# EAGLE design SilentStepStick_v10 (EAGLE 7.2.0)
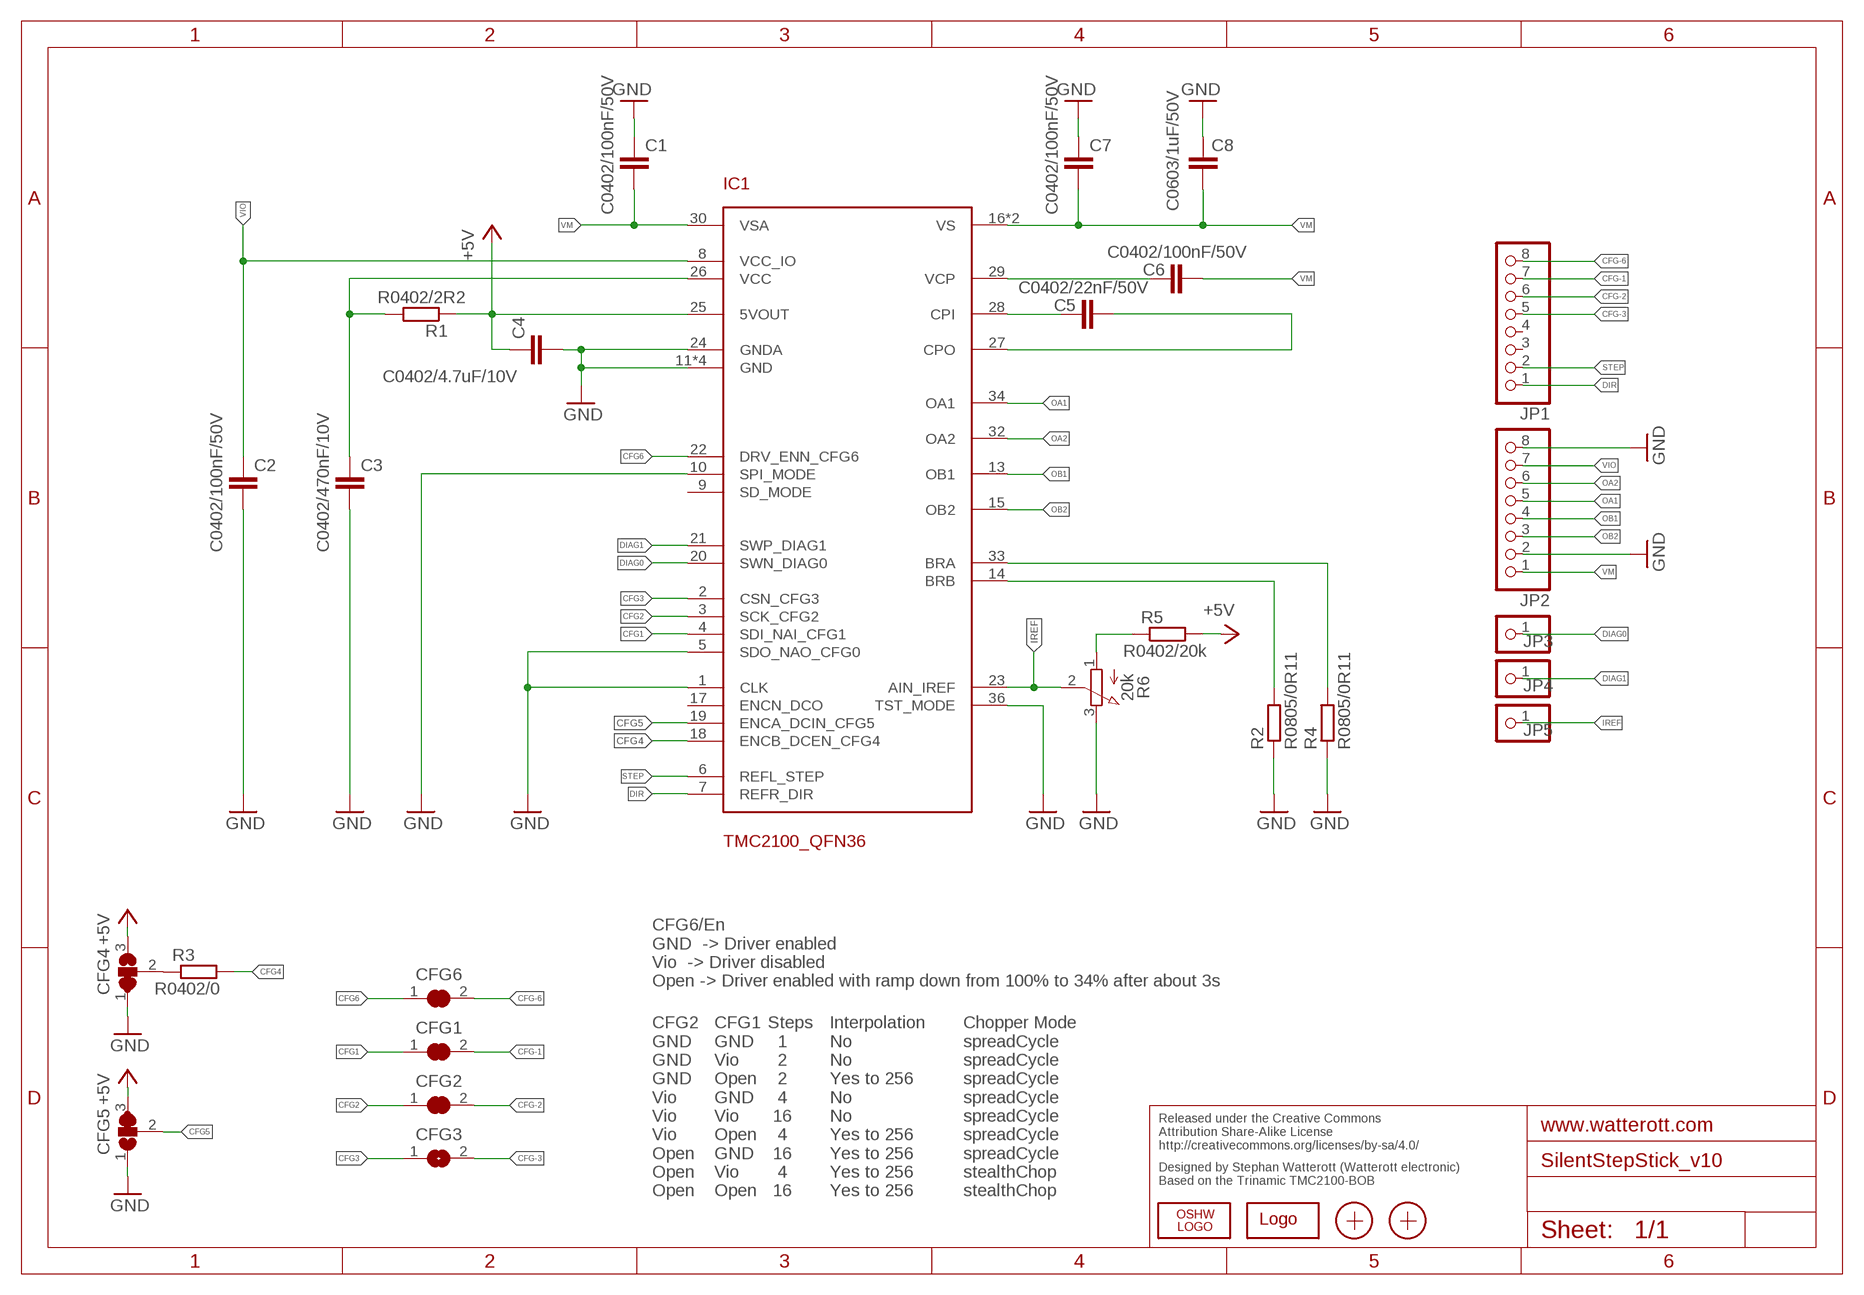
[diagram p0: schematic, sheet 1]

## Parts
C1  C0402/100nF/50V  C-EUC0402  [C0402]
C2  C0402/100nF/50V  C-EUC0402  [C0402]
C3  C0402/470nF/10V  C-EUC0402  [C0402]
C4  C0402/4.7uF/10V  C-EUC0402  [C0402]
C5  C0402/22nF/50V  C-EUC0402  [C0402]
C6  C0402/100nF/50V  C-EUC0402  [C0402]
C7  C0402/100nF/50V  C-EUC0402  [C0402]
C8  C0603/1uF/50V  C-EUC0603  [C0603]
CFG1  JUMPER2-0201  [JUMPER2-0201]
CFG2  JUMPER2-0201  [JUMPER2-0201]
CFG3  JUMPER2-0201  [JUMPER2-0201]
CFG4  JUMPER3-0201-NC  [JUMPER3-0201_NC]
CFG5  JUMPER3-0201  [JUMPER3-0201]
CFG6  JUMPER2-0201  [JUMPER2-0201]
IC1  TMC2100_QFN36  [QFN36]
JP1  PINHD-1X08_2.54-S  [1X08-S]
JP2  PINHD-1X08_2.54-S  [1X08-S]
JP3  PINHD-1X1  [1X01]
JP4  PINHD-1X1  [1X01]
JP5  PINHD-1X1  [1X01]
LOGO1  OSHW_LOGOX0070  [OSHW_6X70]
LOGO2  LOGO-S_PLACE_M  [SPARK_TPLACE_M]
R1  R0402/2R2  R-EU_R0402  [R0402]
R2  R0805/0R11  R-EU_M0805  [M0805]
R3  R0402/0  R-EU_R0402  [R0402]
R4  R0805/0R11  R-EU_M0805  [M0805]
R5  R0402/20k  R-EU_R0402  [R0402]
R6  20k  POTEVM3R  [POT_EVM3R]
X1  PASSER-07  [PASSER_07MM]
X2  PASSER-07  [PASSER_07MM]

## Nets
+5V: C4.1 CFG4.3 CFG5.3 IC1.25(5VOUT) R1.1 R5.2
CFG1: CFG1.1 IC1.4(SDI_NAI_CFG1)
CFG2: CFG2.1 IC1.3(SCK_CFG2)
CFG3: CFG3.1 IC1.2(CSN_CFG3)
CFG4: IC1.18(ENCB_DCEN_CFG4) R3.2
CFG5: CFG5.2 IC1.19(ENCA_DCIN_CFG5)
CFG6: CFG6.1 IC1.22(DRV_ENN_CFG6)
CFG-1: CFG1.2 JP1.7
CFG-2: CFG2.2 JP1.6
CFG-3: CFG3.2 JP1.5
CFG-6: CFG6.2 JP1.8
CPI: C5.1 IC1.28(CPI)
CPO: C5.2 IC1.27(CPO)
DIAG0: IC1.20(SWN_DIAG0) JP3.1
DIAG1: IC1.21(SWP_DIAG1) JP4.1
DIR: IC1.7(REFR_DIR) JP1.1
GND: C1.1 C2.2 C3.2 C4.2 C7.1 C8.2 CFG4.1 CFG5.1 IC1.1(CLK) IC1.5(SDO_NAO_CFG0) IC1.10(SPI_MODE) IC1.11(GND) IC1.12(GND) IC1.24(GNDA) IC1.35(GND) IC1.36(TST_MODE) IC1.GND_PAD(GND) JP2.2 JP2.8 R2.1 R4.1 R6.3(E)
IREF: IC1.23(AIN_IREF) JP5.1 R6.2(S)
N$1: CFG4.2 R3.1
N$7: IC1.33(BRA) R4.2
N$9: IC1.14(BRB) R2.2
OA1: IC1.34(OA1) JP2.5
OA2: IC1.32(OA2) JP2.6
OB1: IC1.13(OB1) JP2.4
OB2: IC1.15(OB2) JP2.3
STEP: IC1.6(REFL_STEP) JP1.2
VCC: C3.1 IC1.26(VCC) R1.2
VCP: C6.1 IC1.29(VCP)
VIO: C2.1 IC1.8(VCC_IO) JP2.7
VM: C1.2 C6.2 C7.2 C8.1 IC1.16(VS) IC1.30(VSA) IC1.31(VS) JP2.1
VREF1: R5.1 R6.1(A)
Unconnected: IC1.9(SD_MODE) IC1.17(ENCN_DCO) JP1.3 JP1.4

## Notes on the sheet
- CFG6/En
  GND  -> Driver enabled
  Vio  -> Driver disabled
  Open -> Driver enabled with ramp down from 100% to 34% after about 3s
- CFG2
  GND
  GND
  GND
  Vio
  Vio
  Vio
  Open
  Open
  Open
- CFG1
  GND
  Vio
  Open
  GND
  Vio
  Open
  GND
  Vio
  Open
- Steps
    1
    2
    2
    4
   16
    4
   16
    4
   16
- Interpolation
  No
  No
  Yes to 256
  No
  No
  Yes to 256
  Yes to 256
  Yes to 256
  Yes to 256
- Chopper Mode
  spreadCycle
  spreadCycle
  spreadCycle
  spreadCycle
  spreadCycle
  spreadCycle
  spreadCycle
  stealthChop
  stealthChop
- Released under the Creative Commons
  Attribution Share-Alike License
  http://creativecommons.org/licenses/by-sa/4.0/
- Designed by Stephan Watterott (Watterott electronic) 
  Based on the Trinamic TMC2100-BOB

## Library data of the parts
C1-C8 = rcl:C-EU: CAPACITOR, European symbol
CFG1-CFG3 CFG6 = we-rcl:JUMPER2: 2 Pin Jumpers
CFG4 CFG5 = we-rcl:JUMPER3: 3 Pin Jumpers
IC1 = TMC2100_QFN:TMC2100_QFN36
JP1 JP2 = pinhead-2:PINHD-1X08: PIN HEADER
JP3-JP5 = pinhead:PINHD-1X1: PIN HEADER
LOGO1 = we-symbol:OSHW_LOGO: Open-Source-Hardware Logo
LOGO2 = we-symbol:LOGO: Watterott electronic Logo
R1-R5 = rcl:R-EU_: RESISTOR, European symbol
R6 = we-rcl:POT: Potentiometer
X1 X2 = we-symbol:PASSER: Fiducial Markers

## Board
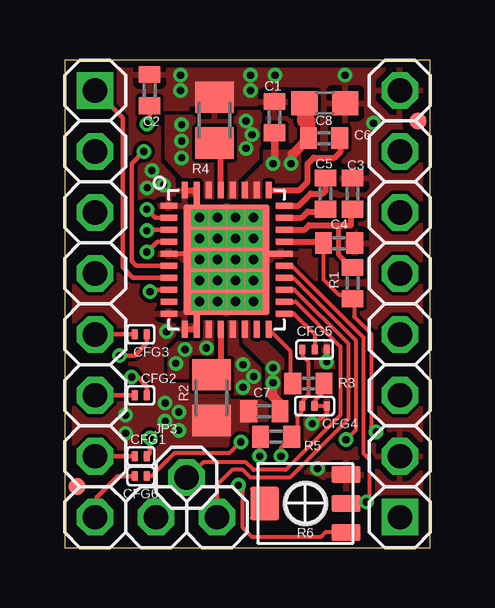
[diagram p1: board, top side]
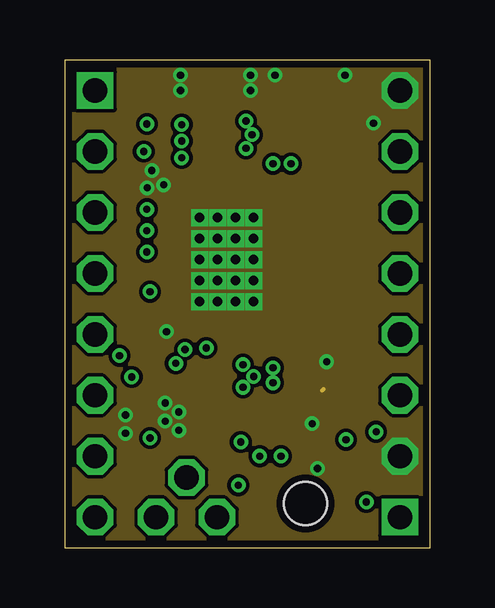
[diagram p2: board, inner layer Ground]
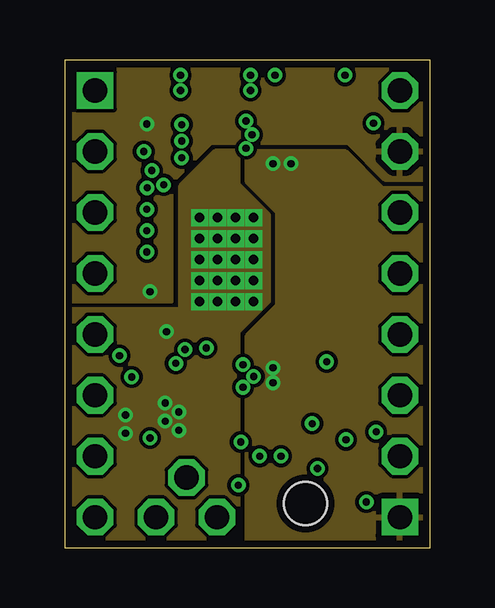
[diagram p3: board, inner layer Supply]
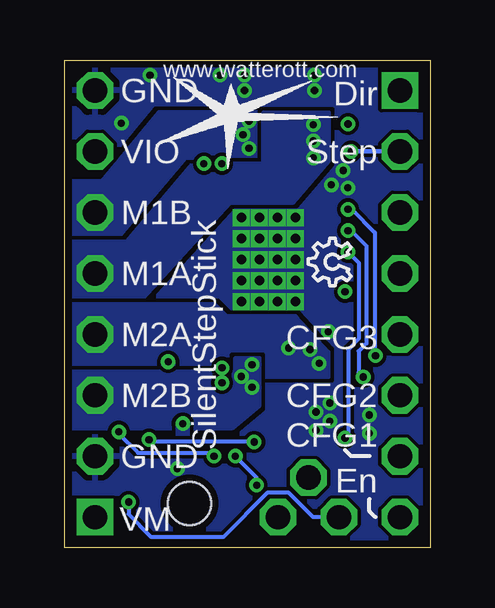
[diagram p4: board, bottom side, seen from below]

Size 15.24 x 20.32 mm. Coordinates in mm from the lower left corner, seen from the top.
Outline: 0,0 15.24,0 15.24,20.32 0,20.32 0,0
Copper layers (1*2*15*16): Top 0.035mm / dielectric 0.36mm / Ground 0.035mm / dielectric 0.71mm / Supply 0.035mm / dielectric 0.2mm / Bottom 0.035mm
Design rules "Default_WE_Euro *": minimum track width 0.15mm, minimum drill 0.25mm, track to track 0.15mm, track to pad 0.15mm, pad to pad 0.15mm, via to via 0.15mm, smd to smd 0mil, copper to edge 0.3mm, drill to drill 8mil, minimum pad ring 10mil, minimum via ring 6mil, stop-mask expansion 2mil, vias tented up to drill 0.35mm, thermal gap 10mil

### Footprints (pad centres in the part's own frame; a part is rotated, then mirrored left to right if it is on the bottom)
C0402 = smd 0.7 x 0.9: 1 -0.65,0; 2 0.65,0
C0603 = smd 1.1 x 1: 1 -0.85,0; 2 0.85,0
JUMPER2-0201 = smd 0.43 x 0.28: 1 0,0.255; 2 0,-0.255
JUMPER3-0201_NC = smd 0.43 x 0.28: 1 0,0.509; 2 0,-0.001; 3 0,-0.509
JUMPER3-0201 = smd 0.43 x 0.28: 1 0,0.51; 2 0,0; 3 0,-0.51
QFN36 = smd 0.7 x 0.25: 1 -2.4,2.25; 2 -2.4,1.75; 3 -2.4,1.25; 4 -2.4,0.75; 5 -2.4,0.25; 6 -2.4,-0.25; 7 -2.4,-0.75; 8 -2.4,-1.25; 9 -2.4,-1.75; 10 -2.4,-2.25; 19 2.4,-2.25; 20 2.4,-1.75; 21 2.4,-1.25; 22 2.4,-0.75; 23 2.4,-0.25; 25 2.4,0.75; 26 2.4,1.25; 27 2.4,1.75; 28 2.4,2.25 | smd 0.25 x 0.7: 11 -1.75,-2.9; 13 -0.75,-2.9; 14 -0.25,-2.9; 15 0.25,-2.9; 16 0.75,-2.9; 17 1.25,-2.9; 18 1.75,-2.9; 29 1.75,2.9; 30 1.25,2.9; 31 0.75,2.9; 32 0.25,2.9; 33 -0.25,2.9; 34 -0.75,2.9; 36 -1.75,2.9 | smd 0.25 x 1: 12 -1.25,-2.75; 35 -1.25,2.75 | smd 1 x 0.25: 24 2.25,0.25 | smd 3.6 x 4.6: GND_PAD 0,0
1X08-S = drill 1.016 square: 1 -8.89,0 | drill 1.016 octagon: 2 -6.35,0; 3 -3.81,0; 4 -1.27,0; 5 1.27,0; 6 3.81,0; 7 6.35,0; 8 8.89,0
1X01 = drill 1.016 octagon: 1 0,0
R0402 = smd 0.7 x 0.9: 1 -0.65,0; 2 0.65,0
M0805 = smd 1.3 x 1.6: 1 -0.95,0; 2 0.95,0
POT_EVM3R = smd 0.7 x 1.2: 1 -1.2,-1.7; 2 0,-1.7; 3 1.2,-1.7 | smd 1.4 x 1.2: MOUNT 0,1.7 | hole 1.8: 0,0
PASSER_07MM = smd 0.7 x 0.7: X 0,0

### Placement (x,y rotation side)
C1  8.75,17.94 270 top
C2  3.55,19.07 90 top
C3  12,14.75 90 top
C4  11.44,12.69 0 top
C5  10.88,14.75 270 top
C6  10.81,17.06 180 top
C7  8.32,5.68 0 top
C8  10.84,18.53 0 top
CFG1  3.17,3.81 270 top
CFG2  3.17,6.35 270 top
CFG3  3.17,8.89 270 top
CFG4  10.41,5.91 270 top
CFG5  10.41,8.26 270 top
CFG6  3.17,2.98 270 top
IC1  6.75,12 0 top
JP1  1.27,10.16 270 top
JP2  13.97,10.16 90 top
JP3  5.08,2.92 0 top
JP4  6.35,1.27 0 top
JP5  3.81,1.27 0 top
LOGO1  3.3,10.92 90 bottom
LOGO2  8.26,18.03 0 bottom
R1  12,11.03 90 top
R2  6.12,6.25 90 top
R3  10.16,6.85 180 top
R4  6.25,17.81 270 top
R5  8.81,4.62 0 top
R6  10.03,1.84 90 top
X1  0.51,2.54 0 top
X2  14.73,17.78 0 top

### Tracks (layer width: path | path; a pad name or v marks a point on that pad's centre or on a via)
+5V  (via drill 0.3 pad 0.41)
  Top 0.16: CFG5.3 9.9,8.32 9.91,8.32 9.91,8 10.16,7.75 10.16,6.36 9.9,6.11 CFG4.3 9.86,5.85 9.86,5.61 9.69,5.45 9.69,4.82 9.66,4.82 R5.2 9.02,4.18 v9.02,3.81 9.02,3.99 | C4.1 10.79,11.18 11.43,10.54 11.75,10.54 | 11.75,10.54 11.84,10.54 R1.1 | 11.75,10.54 12.06,10.22 12.06,9.63 12.78,8.91 12.78,5.03 v12.98,4.83
  Top 0.254: IC1.25 10.79,12.75 C4.1
  Bottom 0.16: v9.02,3.81 9.08,3.87 9.1,3.87 9.17,3.95 12.18,3.95 12.98,4.75 v12.98,4.83
CFG1  (via drill 0.3)
  Top 0.18: IC1.4 3.86,12.75 v3.43,12.32 | v3.56,4.57 3.56,3.94 CFG1.1
  Bottom 0.16: v3.43,12.32 2.98,11.87 2.98,8.7 3.43,8.26 3.43,4.7 v3.56,4.57
CFG2  (via drill 0.3)
  Top 0.16: 3.6,13.25 3.47,13.25 v3.43,13.21
  Top 0.18: IC1.3 3.6,13.25 | v2.8,7.11 3.05,7.11 3.43,6.73 CFG2.1
  Bottom 0.16: v3.43,13.21 3.3,13.21 2.67,12.57 2.67,8.51 2.99,8.19 2.99,7.3 v2.79,7.11 v2.8,7.11
CFG3  (via drill 0.3)
  Top 0.18: IC1.2 3.78,13.75 v3.43,14.1 | v2.29,8 2.92,8 3.43,8.51 CFG3.1
  Bottom 0.16: v3.43,14.1 3.28,14.1 2.31,13.12 2.31,8.06 2.29,8.04 v2.29,8
CFG4
  Top 0.16: IC1.18 9.4,8.2 9.4,6.96 R3.2
CFG5
  Top 0.16: IC1.19 9.55,9.75 10.41,8.89 CFG5.2
CFG6  (via drill 0.3 pad 0.41)
  Top 0.16: IC1.22 9.53,11.24 12.13,8.64 12.13,4.9 v11.72,4.5 | CFG6.1 3.62,2.98 4.57,3.94 6.87,3.94 v7.34,4.41
  Bottom 0.16: v7.34,4.41 11.63,4.41 v11.72,4.5
CFG-1
  Top 0.18: CFG1.2 JP1.7
CFG-2
  Top 0.18: CFG2.2 JP1.6
CFG-3
  Top 0.18: CFG3.2 JP1.5
CFG-6
  Top 0.18: JP1.8 1.33,1.33 1.33,2.1 2.22,2.98 CFG6.2
CPI
  Top 0.254: IC1.28 9.75,14.25 10.25,14.75 10.75,14.75 10.88,14.88 C5.1
CPO
  Top 0.254: IC1.27 9.88,13.75 10.12,14 10.78,14 C5.2
DIAG0
  Top 0.16: IC1.20 9.63,10.25 11.49,8.38 11.49,5.52 9.21,3.24 7.87,3.24 7.56,3.56 5.78,3.56 5.46,3.24 5.14,2.92 JP3.1
DIAG1
  Top 0.16: IC1.21 9.57,10.75 11.81,8.51 11.81,5.36 9.37,2.92 7.75,2.92 7.43,3.24 6.99,3.24 6.35,2.6 JP4.1
DIR
  Top 0.18: IC1.7 2.85,11.25 2.41,11.68 2.41,17.91 JP1.1
GND  (via drill 0.3, 0.4, 0.4 pad 0.41)
  Top 0.16: CFG4.1 10.92,5.59 10.73,5.4 10.67,5.4 10.6,5.33 | v10.92,7.75 CFG5.1
  Top 0.18: IC1.5 5.38,12.25 v5.62,12
  Top 0.254: IC1.11 5.35,9.1 IC1.12 | IC1.36 5.35,14.9 IC1.35 | IC1.24 8.12,12.25 v7.88,12
  Ground 0.16: 10.79,6.6 10.73,6.54
  other vias: 4.83,19.68 4.83,19.05 7.75,19.05 4.76,5.65 4.19,6.03 4.19,5.27 4.25,9 5.62,13.75 6.38,13.75 7.12,13.75 7.88,13.75 5.62,12.88 6.38,12.88 7.12,12.88 7.88,12.88 6.38,12 7.12,12 6.38,11.12 5.62,11.12 7.12,11.12 7.88,11.12 5.62,10.25 6.38,10.25 7.12,10.25 7.75,19.68 12.88,17.69 8.76,19.68 4.13,15.12 3.63,15.72 7.88,10.25 10.31,5.17 4.76,4.89 3.44,15 11.68,19.68 2.54,5.52 2.54,4.76 10.54,3.3
  pour Top (rank 6): 0,20.32 15.24,20.32 15.24,0 0,0
  pour Ground (no thermals): 0,20.32 15.24,20.32 15.24,0 0,0
  pour Bottom (rank 6): 0,20.32 15.24,20.32 15.24,0 0,0
  pour Top (no thermals): 5.25,18.5 7.25,18.5 7.25,20.12 5.25,20.12
  pour Top (no thermals): 5,4.25 8.2,4.25 8.2,6.07 5,6.07
  pour Supply: 6.29,16.51 4.83,15.05 4.83,9.91 0,9.91 0,0 7.24,0 7.24,9.02 8.51,10.29 8.51,13.84 7.24,15.11 7.24,16.51
IREF  (via drill 0.3)
  Top 0.16: 9.47,11.75 IC1.23 9.22,11.68 9.53,11.68 12.45,8.76 12.45,3.94 12.7,3.68 12.7,2.16 12.45,1.91 | 11.77,1.88 R6.2 | 11.62,1.97 11.67,1.91 R6.2 | 12.45,1.91 11.8,1.91 R6.2 | 12.45,1.91 v12.57,1.91
  Bottom 0.16: JP5.1 4.89,1.27 5.91,2.29 6.79,2.29 8.64,0.45 11.62,0.45 12.57,1.4 v12.57,1.91
N$1
  Top 0.16: 10.86,7.1 10.86,7.05 | 10.86,7.05 10.86,6.57 10.41,6.12 CFG4.2 | R3.1 10.81,7.1 10.86,7.05
N$7
  Top 0.254: IC1.33 6.5,16.61 R4.2
N$9
  Top 0.254: IC1.14 6.5,7.58 R2.2
N$10
  Top 0.16: 10.41,5.91 10.92,5.91
OA1  (via drill 0.3)
  other vias: 4.88,17.63 4.88,16.24 4.88,16.94
  pour Top (rank 2, no thermals): 6.25,14.62 6.25,16.12 5.38,16.12 5.38,17.94 4.25,17.94 4.25,16.25 5.06,15.38 5.88,15.38 5.88,14.62
  pour Bottom (rank 3, no thermals): 12.25,10.12 15.25,10.12 15.25,12.75 12.62,12.75 9.88,16 6.94,16 6.94,18.12 4.25,18.12 4.25,16.12 5.75,14.38 8.37,14.38
OA2  (via drill 0.3)
  other vias: 7.81,17.21 7.56,16.64 7.56,17.78
  pour Top (rank 3, no thermals): 8.12,14.62 8.12,18.12 7.12,18.12 7.12,16.12 6.75,16.13 6.75,14.62
  pour Bottom (rank 4, no thermals): 15.25,13 12.62,13 9.88,16.12 7.12,16.12 7.12,18.13 11.31,18.13 13.69,15.25 15.25,15.25
OB1  (via drill 0.3)
  other vias: 5.02,8.26 5.91,8.32 4.64,7.68
  pour Top (rank 2, no thermals): 6.31,7.14 6.31,9.38 5.75,9.38 5.75,8.5 4.75,8.5 4.38,8.12 4.38,7.14
  pour Bottom (rank 2, no thermals): 15.25,10.12 15.19,7.62 8.4,7.62 8.34,8.12 7,8.12 7,7.14 4.25,7.14 4.25,8.12 5.62,9.62 8.5,9.62 9,10.12
OB2  (via drill 0.3)
  other vias: 7.43,7.62 7.88,7.13 7.43,6.68
  pour Top (rank 3, no thermals): 8.25,6.44 8.25,9.38 6.5,9.38 6.5,6.44
  pour Bottom (no thermals): 15.25,7.31 15.25,5 8.25,5 7.12,5.94 7.12,7.87 8.13,7.87 arc11 8.15,7.31
STEP  (via drill 0.3)
  Top 0.18: IC1.6 2.98,11.75 2.79,11.94 2.79,16 v3.3,16.51
  Bottom 0.18: v3.3,16.51 JP1.2
VCC
  Top 0.16: 11.94,11.68 11.95,11.68 R1.2
  Top 0.2: 11.94,11.68 11.43,12.19 11.43,13.31 11.56,13.44
  Top 0.254: IC1.26 10,13.25 10.19,13.44 11.56,13.44 11.94,13.44 11.94,14.04 C3.1 11.88,13.97
VCP
  Top 0.254: IC1.29 9.78,14.9 10.12,15.25 10.12,16 10.38,16.25 11.25,16.25 11.5,16.5 11.5,17.02 C6.1
VIO  (via drill 0.3)
  Top 0.16: 3.55,17.9 3.55,17.77 v3.43,17.65
  Top 0.18: C2.1 3.55,17.9 | IC1.8 3.64,10.75 v3.56,10.67
  Supply 0.18: v3.56,10.67 3.43,10.54
  pour Supply: 15.24,15.36 15.24,20.32 0,20.32 0,10.29 4.45,10.29 4.45,15.24 6.1,16.89 11.81,16.88 13.34,15.36
VM  (via drill 0.3)
  Top 0.305: C1.2 8.75,16.06 v8.69,16 | v9.44,16 9.44,16.31 9.5,16.38
  Top 0.406: 9.5,16.4 C6.2 | v8.68,6.87 8.72,6.84 8.64,6.75 8.64,6.35 8.97,6.01 C7.2
  Top 0.61: C6.2 10.16,17.78 9.99,17.78 C8.1
  other vias: 8.68,7.49
  pour Top (no thermals): 7.5,14.62 7.5,15.12 8.38,16 8.38,16.5 9.75,16.5 9.75,15 9.38,14.62
  pour Top (no thermals): 7.5,9.38 7.5,8.62 8.44,7.69 8.44,6.44 9.06,6.44 9.06,7.81 8,8.88 8,9.38
  pour Supply: 15.24,0 7.62,0 7.62,8.83 8.89,10.1 8.89,13.97 7.62,15.24 7.62,16.51 11.68,16.51 13.21,14.99 15.24,14.99
VREF1  (via drill 0.3)
  Top 0.16: 8.37,4.64 8.28,4.56 8.23,4.56 R5.1 | v8.13,3.81 8.13,4.59 | R6.1 10.87,0.64 10.67,0.45 7.81,0.45 7.43,0.83 7.43,2.41 v7.24,2.6
  Top 0.18: 8.13,4.59 R5.1
  Bottom 0.16: v7.24,2.6 7.24,2.92 v8.13,3.81

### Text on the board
bPlace: www.watterott.com | Dir | GND | Step | VIO | M1B | M1A | CFG3 | M2A | CFG2 | M2B | CFG1 | SilentStepStick | En | GND | VM
Document: Dir | GND | Step | Vio - 3.3-5V | nc | Motor Coil 1-B | nc | Motor Coil 1-A | CFG3 | Motor Coil 2-A | CFG2 | Motor Coil 2-B | CFG1 | GND | En/CFG6 | Vm | VRef | DIAG0 | DIAG1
